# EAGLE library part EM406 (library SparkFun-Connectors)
EM406 GPS Connector Here is a six pin vertical 1.0mm pitch connector. It is useful if you need something very tiny as a connection. These are not the standard JST type connectors we use on most of our boards, but are actually the much smaller JST-SH type. Here is the connector we sell at SparkFun: JST SH Vertical 6-Pin Connector - SMD (GPS-00579) Datasheet It was used on these SparkFun products: SparkFun GPS Breakout (BOB-11818) SparkFun Weather Shield (DEV-12081) And many, many other GPS related products.
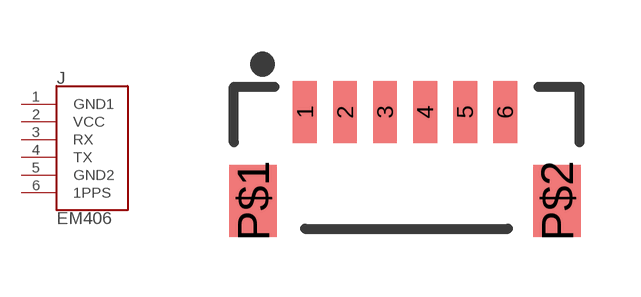
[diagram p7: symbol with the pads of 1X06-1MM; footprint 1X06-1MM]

Designator prefix J

## EM406 (PROD_ID: CONN-08249; SF_ID: GPS-00579)  [1X06-1MM]
1  GND1
2  VCC
3  RX
4  TX
5  GND2
6  1PPS

## Footprint 1X06-1MM (pad centres in mm)
JST SH Vertical 6-Pin Connector -SMD Specifications: Pin count:6 Pin pitch:1mm Datasheet referenced for footprint Example device(s): CONN_06 EM-406
smd 0.6 x 1.55: 1 -2.54,1.27; 2 -1.54,1.27; 3 -0.54,1.27; 4 0.46,1.27; 5 1.46,1.27; 6 2.46,1.27
smd 1.2 x 1.8: P$1 -3.84,-0.955; P$2 3.76,-0.955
